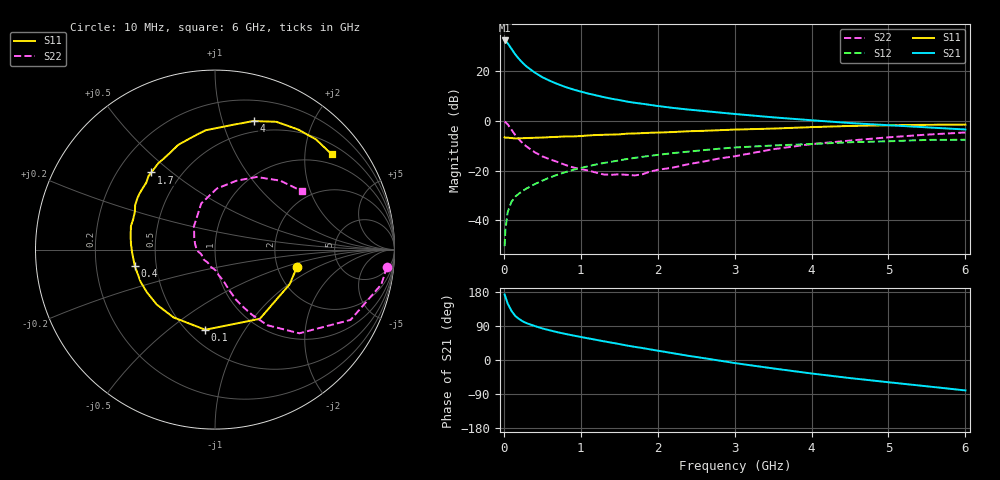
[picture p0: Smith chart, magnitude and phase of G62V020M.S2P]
! SIEMENS Small Signal Semiconductors
! BFG193
! Si NPN RF Bipolar Junction Transistor in SOT223
! VCE = 2 V  IC = 20 mA
! Common Emitter S-Parameters:  August  1996
# GHz  S  MA  R  50
!  f  S11  S21  S12  S22
! GHz  MAG  ANG  MAG  ANG  MAG  ANG  MAG  ANG
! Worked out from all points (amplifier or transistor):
!   36 points, 10 MHz to 6 GHz, reference 50 ohm
!   highest |S21| = 32.4 dB at 10 MHz (marker M1)
!   |S21| within 3 dB of that: start of sweep to 91.5 MHz
!   unconditionally stable (mu >= 1): 669 MHz to 2.64 GHz
!   at 250 MHz: K = 0.75, MSG = 25.6 dB, |S12| = -28.1 dB
!   at 1.4 GHz: K = 1.06, MAG = 11.2 dB, |S12| = -16.4 dB
!   at 6 GHz: K = 0.92, MSG = 2.1 dB, |S12| = -7.6 dB
!   S11 on the Smith chart (normalised r, x): 10 MHz: 2.56, -0.65; 100 MHz: 0.61, -0.68; 400 MHz: 0.38, -0.09; 1.7 GHz: 0.34, +0.43; 4 GHz: 0.39, +1.27; 6 GHz: 0.73, +2.63
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0.01  0.4666 -12.2  41.57 172.9  0.003 86.2  0.9624 -5.8
0.02  0.4587 -24.9  40.81 167.1  0.0063 82.2  0.947 -11.8
0.05  0.4593 -57.0  36.47 148.9  0.0146 69.4  0.8509 -27.4
0.1  0.45 -96.9  28.16 129.5  0.0237 61.9  0.6618 -44.8
0.15  0.4429 -121.5  21.62 115.9  0.0299 56.8  0.5136 -55.2
0.2  0.4462 -136.6  17.45 107.9  0.0346 57.5  0.4194 -60.3
0.25  0.4478 -147.9  14.38 101.5  0.0394 56.5  0.3465 -64.5
0.3  0.4515 -156.4  12.26 96.8  0.0439 57.9  0.3011 -67.3
0.4  0.4564 -168.3  9.42 89.8  0.0531 58.7  0.2344 -71.0
0.5  0.4614 -177.4  7.577 83.3  0.0625 59.0  0.1929 -73.7
0.6  0.47 175.7  6.384 78.2  0.0727 59.1  0.168 -76.7
0.7  0.4769 170.2  5.503 73.2  0.0826 58.5  0.1483 -80.9
0.9  0.4862 159.6  4.299 64.7  0.1032 56.3  0.1155 -88.5
1.1  0.5094 150.8  3.538 57.0  0.1223 53.4  0.1 -102.5
1.4  0.5294 138.9  2.788 45.8  0.1506 47.9  0.0821 -127.9
1.7  0.5578 129.6  2.313 34.8  0.1798 42.1  0.0797 -156.8
2.2  0.5958 114.5  1.821 17.9  0.2245 30.9  0.1147 164.9
3.5  0.6992 82.6  1.178 -22.2  0.3194 0.2  0.2684 106.6
4  0.748 73.3  1.029 -35.6  0.3422 -9.5  0.3404 88.2
4.5  0.79 64.3  0.904 -47.7  0.3709 -19.5  0.4015 72.8
5.5  0.8329 47.4  0.74 -69.4  0.4133 -42.6  0.5288 46.6
6  0.8393 39.2  0.67 -80.3  0.4166 -55.7  0.5832 34.0
